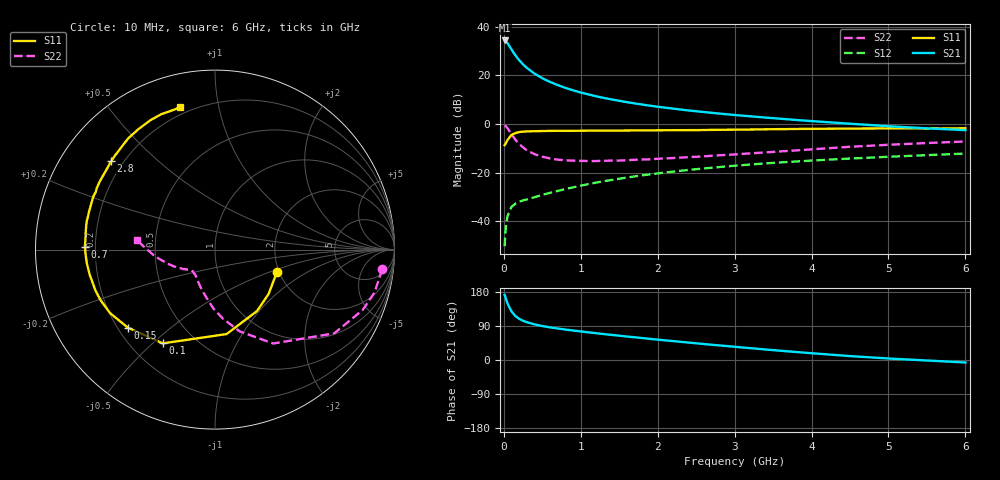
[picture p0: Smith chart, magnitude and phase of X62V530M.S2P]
! SIEMENS Small Signal Semiconductors
! BFP193W
! Si NPN RF Bipolar Junction Transistor in SOT343
! VCE = 2.5 V  IC = 30 mA
! Common Emitter S-Parameters:  April 1994
# GHz  S  MA  R  50
!  f  S11  S21  S12  S22
! GHz  MAG  ANG  MAG  ANG  MAG  ANG  MAG  ANG
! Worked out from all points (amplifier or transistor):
!   40 points, 10 MHz to 6 GHz, reference 50 ohm
!   highest |S21| = 34.3 dB at 10 MHz (marker M1)
!   |S21| within 3 dB of that: start of sweep to 85.71 MHz
!   unconditionally stable (mu >= 1): 758.3 MHz to 3.987 GHz
!   at 200 MHz: K = 0.45, MSG = 29.0 dB, |S12| = -31.9 dB
!   at 1.5 GHz: K = 1.13, MAG = 13.8 dB, |S12| = -22.5 dB
!   at 6 GHz: K = 0.94, MSG = 4.8 dB, |S12| = -12.1 dB
!   lowest NFmin = 1.90 dB at 450 MHz
!   S11 on the Smith chart (normalised r, x): 10 MHz: 1.94, -0.56; 100 MHz: 0.33, -0.54; 150 MHz: 0.24, -0.36; 700 MHz: 0.16, +0.01; 2.8 GHz: 0.15, +0.36; 6 GHz: 0.16, +0.77
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0.01  0.3669 -20.0  51.95 172.2  0.0031 86.1  0.9381 -6.7
0.02  0.3874 -39.4  51.18 166.2  0.0059 75.9  0.9202 -15.1
0.03  0.4148 -55.6  49.69 159.8  0.0087 76.6  0.8891 -22.2
0.05  0.475 -82.2  45.21 148.1  0.0132 63.8  0.8117 -35.1
0.1  0.5978 -119.1  33.87 128.2  0.0199 50.2  0.6156 -58.2
0.15  0.6517 -138.1  25.72 116.1  0.0232 43.8  0.476 -73.2
0.2  0.6834 -148.8  20.33 108.7  0.0254 41.4  0.3869 -83.5
0.25  0.6972 -156.2  16.78 103.5  0.027 41.9  0.3305 -91.2
0.3  0.7039 -161.2  14.13 99.8  0.0283 42.8  0.2873 -97.5
0.4  0.7119 -168.7  10.79 93.9  0.0315 44.7  0.2398 -107.0
0.5  0.7179 -173.7  8.722 89.6  0.035 47.9  0.2131 -114.2
0.6  0.7209 -177.5  7.297 86.1  0.0386 50.1  0.1962 -119.9
0.7  0.7257 178.9  6.314 83.1  0.0422 52.2  0.1856 -124.1
0.9  0.7253 173.8  4.916 77.8  0.05 55.1  0.1769 -130.4
1.1  0.73 169.5  4.05 73.0  0.0584 56.9  0.1734 -134.8
1.6  0.7355 159.7  2.814 61.9  0.0796 58.2  0.1803 -140.8
2.2  0.7458 149.4  2.068 49.9  0.1054 56.6  0.1999 -147.2
2.8  0.76 139.7  1.639 38.5  0.1306 53.3  0.2281 -153.1
3.2  0.7702 133.6  1.441 31.3  0.147 50.8  0.2492 -158.1
4.5  0.8055 116.6  1.013 10.3  0.1952 41.6  0.3404 -174.3
5.5  0.8109 108.0  0.815 -1.3  0.2294 35.1  0.4066 176.5
6  0.8163 103.8  0.748 -6.6  0.2472 32.1  0.4379 172.9
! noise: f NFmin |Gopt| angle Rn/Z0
0.45  1.9  0.4  180  0.09
0.9  1.95  0.43  -173  0.11
1.8  2.4  0.58  -144  0.24
